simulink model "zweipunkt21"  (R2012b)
settings: Solver=ode45  StartTime=0.0  StopTime=10.0  RelTol=1e-3
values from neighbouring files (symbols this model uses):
  hy = 0.01    [fuellstnd_3.m]    (also in fuellstnd_31.m; regulator_1.m = 2; zweipunkt_1.m = 20; zweipunkt_2.m = 0)
  Kp = 10    [zweipunkt_1.m]    (also in zweipunkt_2.m; zweipunkt_21.m; zweipunkt_31.m; zweipunkt_32.m = 1)
  T1 = 1    [PID_windup1.m]    (also in pol_1.m = -5; pol_2.m = -5; pol_3.m = -5; sprung.m = x(2))
  T2 = 5    [PID_windup1.m]    (also in pol_1.m = 10; pol_2.m = 10; pol_3.m = 10; sprung.m = x(3))
  T3 = 10    [PID_windup1.m]    (also in sprung.m = x(4); sprung_1.m = x(4); zweipunkt_21.m = 20; zweipunkt_31.m = 100)
  ysoll = y.signals.values(:,2)    [ohne_kalman_1.m]    (also in zweipunkt_1.m = 500; zweipunkt_2.m = 500; zweipunkt_21.m = 500; zweipunkt_31.m = 500)

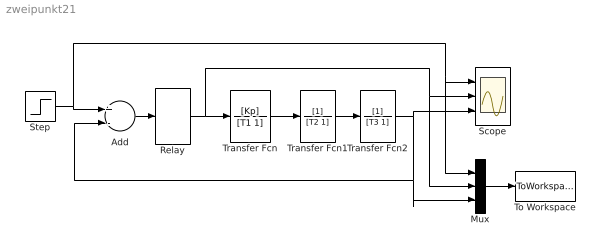
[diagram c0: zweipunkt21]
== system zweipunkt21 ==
  Add : Sum  Inputs=+-
  Mux : Mux  Inputs=3
  Relay : Relay  OnSwitchValue=hy  OffSwitchValue=-hy  OnOutputValue=Ustell  ZeroCross=off
  Scope : Scope  NumInputPorts=3
  Step : Step  Time=10  After=ysoll  SampleTime=0
  To Workspace : ToWorkspace  VariableName=y  SampleTime=-1  SaveFormat=Structure With Time
  Transfer Fcn : TransferFcn  Numerator=[Kp]  Denominator=[T1 1]
  Transfer Fcn1 : TransferFcn  Denominator=[T2 1]
  Transfer Fcn2 : TransferFcn  Denominator=[T3 1]
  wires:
  Add/1 -> Relay/1
  Transfer Fcn/1 -> Transfer Fcn1/1
  Step/1 -> Mux/1, Scope/1, Add/1
  Relay/1 -> Mux/2, Scope/2, Transfer Fcn/1
  Mux/1 -> To Workspace/1
  Transfer Fcn1/1 -> Transfer Fcn2/1
  Transfer Fcn2/1 -> Scope/3, Mux/3, Add/2
